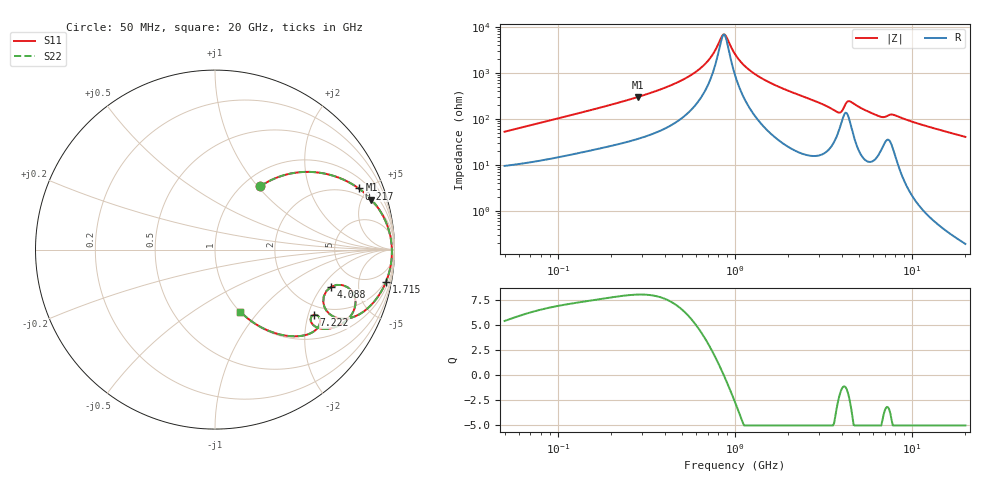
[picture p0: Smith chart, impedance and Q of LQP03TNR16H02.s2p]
!Murata Part Number: LQP03TNR16H02
!These Parameters are Measured in Series Mode Connection
!  o--[Z]--o
!Port1  Port2
!  o-------o
!Freq. Start=50[MHz] Stop=20[GHz], 401[Steps]
# Hz S RI R 50
!Freq.(Hz) S11(Real) S11(Imag) S21(Real) S21(Imag) S12(Real) S12(Imag) S22(Real) S22(Imag)
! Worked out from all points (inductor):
!   401 points, 50 MHz to 20 GHz, reference 50 ohm
!   read as one part in series: L = 162 nH near 51.52 MHz
!   highest Q = 8.07 at 284.2 MHz (marker M1), where L = 166 nH
!   self-resonance near 860.9 MHz
!   S11 on the Smith chart (normalised r, x): 50 MHz: 1.19, +1.03; 217 MHz: 1.56, +4.37; 1.715 GHz: 2, -10; 4.088 GHz: 3.19, -2.47; 7.222 GHz: 1.70, -2.19; 20 GHz: 1.00, -0.81
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5e7  0.2519 0.3518  0.7481 -0.3518  0.7481 -0.3518  0.2519 0.3518
1.364002e8  0.6367 0.4176  0.3633 -0.4176  0.3633 -0.4176  0.6367 0.4176
2.170075e8  0.8009 0.3409  0.1991 -0.3409  0.1991 -0.3409  0.8009 0.3409
2.841629e8  0.8715 0.2784  0.1285 -0.2784  0.1285 -0.2784  0.8715 0.2784
3.721004e8  0.9229 0.2106  0.0771 -0.2106  0.0771 -0.2106  0.9229 0.2106
6.380365e8  0.9769 0.0749  0.0231 -0.0749  0.0231 -0.0749  0.9769 0.0749
7.30116e8  0.9824 0.0418  0.0176 -0.0418  0.0176 -0.0418  0.9824 0.0418
8.608917e8  0.9855 0.0013  0.0145 -0.0013  0.0145 -0.0013  0.9855 0.0013
9.00459e8  0.9857 -0.00979  0.0143 0.00979  0.0143 0.00979  0.9857 -0.00979
1e9  0.9851 -0.0359  0.0149 0.0359  0.0149 0.0359  0.9851 -0.0359
1.23331e9  0.9788 -0.0894  0.0212 0.0894  0.0212 0.0894  0.9788 -0.0894
1.714689e9  0.9525 -0.1799  0.0475 0.1799  0.0475 0.1799  0.9525 -0.1799
2.728004e9  0.8532 -0.3248  0.1468 0.3248  0.1468 0.3248  0.8532 -0.3248
3.572216e9  0.6862 -0.3824  0.3138 0.3824  0.3138 0.3824  0.6862 -0.3824
4.087748e9  0.6457 -0.2083  0.3543 0.2083  0.3543 0.2083  0.6457 -0.2083
4.34015e9  0.7593 -0.2274  0.2407 0.2274  0.2407 0.2274  0.7593 -0.2274
4.608136e9  0.7817 -0.3098  0.2183 0.3098  0.2183 0.3098  0.7817 -0.3098
5.769027e9  0.6456 -0.4384  0.3544 0.4384  0.3544 0.4384  0.6456 -0.4384
7.222371e9  0.553 -0.363  0.447 0.363  0.447 0.363  0.553 -0.363
7.442007e9  0.5753 -0.3701  0.4247 0.3701  0.4247 0.3701  0.5753 -0.3701
1.004137e10  0.4268 -0.4827  0.5732 0.4827  0.5732 0.4827  0.4268 -0.4827
2e10  0.1413 -0.3459  0.8587 0.3459  0.8587 0.3459  0.1413 -0.3459
